PROGRAM MAIN

VAR CONSTANT
	cInitParsResultBuffer	: ST_MA_MultiArray_InitPars :=(eTypeCode := eMA_TypeCode_LREAL, nDims := 2, aDimSizes := [cMaxChannels, cBufferLength]); // buffer length	
END_VAR

VAR
	nInputSelection			: UDINT := 1;														// select input, 0: hardware, 1: function generator
	nChnIdx, i				: UDINT;															// channel index
	nSample					: UDINT;															// current sample
	
	aEl3632 AT %I*			: ARRAY [1..cMaxChannels] OF ARRAY [1..cOversamples] OF INT;		// connect sensor signal here	
	aBuffer					: ARRAY [1..cMaxChannels] OF ARRAY [1..cOversamples] OF LREAL;		// local buffer

	// Source and sink data
	fbSource				: FB_CMA_Source := (stInitPars := cInitParsResultBuffer, nOwnID := eID_Source, aDestIDs := [eID_Spectrum]);																		
	fbSink					: FB_CMA_Sink := (nOwnID := eID_Sink);
	bNewResults				: BOOL;
					
	// generation of signal				
	fbFunctionGenerator		: ARRAY[1..cMaxChannels] OF FB_FunctionGenerator;					// function generator for tests											
	fSetFrequency			: ARRAY[1..cMaxChannels] OF LREAL := [50, 500, 1200, 1400, 3500]; 	// Hz
	fSetAmplitude			: ARRAY[1..cMaxChannels] OF LREAL := [5, 7, 3, 9, 2]; 				// peak amplitude
	
	// RMS computation
	fSumChannels			: LREAL;
	aRmsValue 				: ARRAY [1..cMaxChannels] OF LREAL;									// RMS value for each input channel				
	aSpectrumResult			: ARRAY [1..cMaxChannels] OF ARRAY [1..cFFTResult] OF LREAL; 		// spectrum values for each input channel
	
	// Error history
	fbErrHist				: FB_HRErrHist; // error monitoring
	
END_VAR

// Collect data for each channel.
FOR nChnIdx :=1 TO cMaxChannels DO
	
	// Select source of input.
	CASE nInputSelection OF
		0:  (* input from EL3632 *)
			FOR nSample := 1 TO cOversamples DO
				aBuffer[nChnIdx][nSample] := INT_TO_LREAL(aEl3632[nChnIdx][nSample]);
			END_FOR
			
		1:  (* signal generator *)	
			fbFunctionGenerator[nChnIdx](	bEnable		:= TRUE,
											fFrequency 	:= fSetFrequency[nChnIdx],
											fAmplitude 	:= fSetAmplitude[nChnIdx],											
											eFunction 	:= E_FunctionType.Sine,
											aSignal		:= aBuffer[nChnIdx] );
	END_CASE
END_FOR

// Invalidate input signal on channel 4.
IF bInvalidateCh4 THEN
	FOR i := 1 TO cOversamples DO
		aBuffer[4][i] := F_MA_GetNAN();	
	END_FOR
END_IF

// Collect input data in source.
fbSource.Input2DStd(	pDataIn			:= ADR(aBuffer),
						nDataInSize		:= SIZEOF(aBuffer),
						eElementType	:= eMA_TypeCode_LREAL,
						nOptionPars		:= cCMA_Option_MarkInterruption );										
IF fbSource.bError THEN
	fbErrHist.AddError(bErr:=TRUE, hrErrCode:=fbSource.hrErrorCode, sErrSource:='MAIN.fbSource'); // error monitoring
	//ToDo: if error
END_IF	

// Push results to sink.
fbSink.Output2DStd(		pDataOut 		:= ADR(aSpectrumResult), 
						nDataOutSize 	:= SIZEOF(aSpectrumResult),
						eElementType 	:= eMA_TypeCode_LREAL,
						nOptionPars		:= 0,
						bNewResult		=> bNewResults);		
IF fbSink.bError THEN
	fbErrHist.AddError(bErr:=TRUE, hrErrCode:=fbSink.hrErrorCode, sErrSource:='MAIN.fbSink'); // error monitoring
	// ToDo: if error		
END_IF

// Computation of RMS value.
IF bNewResults THEN
	FOR nChnIdx := 1 TO cMaxChannels DO
		// Calculate RMS value for each channel
		fSumChannels := 0;
		FOR i := 1 TO cFFTResult DO
			fSumChannels := fSumChannels + (aSpectrumResult[nChnIdx][i] * aSpectrumResult[nChnIdx][i]);
		END_FOR
		aRmsValue[nChnIdx] := SQRT(fSumChannels/2);
	END_FOR
	
	// ToDo: Tasks to perform after results for each input channel are available.

END_IF

END_PROGRAM
